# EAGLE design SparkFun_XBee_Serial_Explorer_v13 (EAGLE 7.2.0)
Assembly variants: Attributes
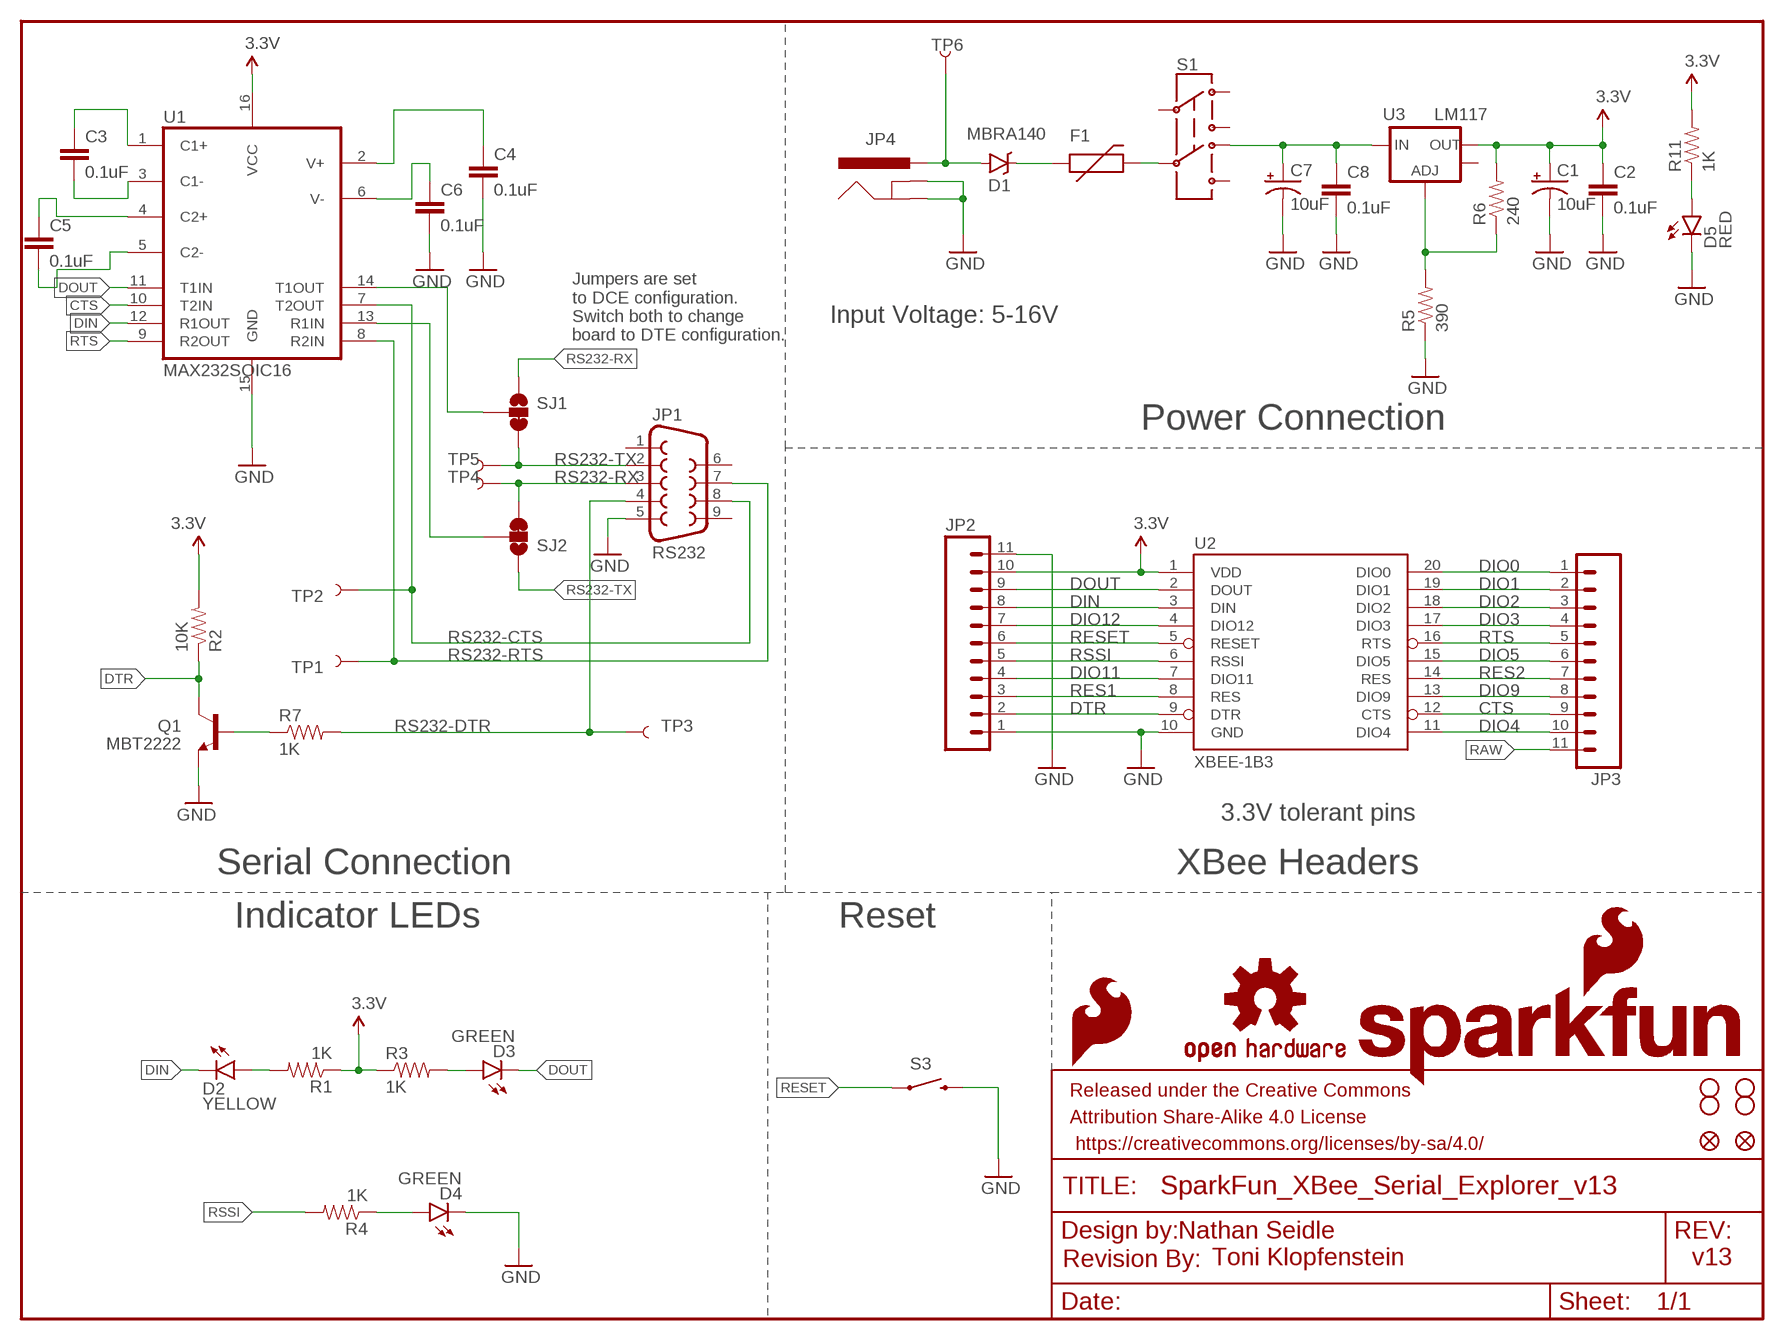
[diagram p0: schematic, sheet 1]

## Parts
C1  10uF  10UF-16V-10%(TANT)  [EIA3216]
C2  0.1uF  0.1UF-25V(+80/-20%)(0603)  [0603-CAP]
C3  0.1uF  0.1UF-25V(+80/-20%)(0603)  [0603-CAP]
C4  0.1uF  0.1UF-25V(+80/-20%)(0603)  [0603-CAP]
C5  0.1uF  0.1UF-25V(+80/-20%)(0603)  [0603-CAP]
C6  0.1uF  0.1UF-25V(+80/-20%)(0603)  [0603-CAP]
C7  10uF  10UF-16V-10%(TANT)  [EIA3216]
C8  0.1uF  0.1UF-25V(+80/-20%)(0603)  [0603-CAP]
D1  MBRA140  DIODE-SCHOTTKY-MBRA140  [SMA-DIODE]
D2  YELLOW  LED-YELLOWLARGE  [LED-1206]
D3  GREEN  LED-GREENLARGE  [LED-1206]
D4  GREEN  LED-GREENLARGE  [LED-1206]
D5  RED  LED-RED1206  [LED-1206]
F1  PTCTHERMISTOR1206  [PTC-1206]
FRAME1  FRAME-LETTER  [CREATIVE_COMMONS]
JP1  RS232  DB9FEMALE  [DB9]
JP2  M11PTH  [1X11]
JP3  M11PTH  [1X11]
JP4  POWER_JACKPTH_LOCK  [POWER_JACK_PTH_LOCK]
LOGO1  OSHW-LOGOL  [OSHW-LOGO-L]
LOGO2  SFE_LOGO_NAME_FLAME.2_INCH  [SFE_LOGO_NAME_FLAME_.2]
LOGO3  SFE_LOGO_FLAME.1_INCH  [SFE_LOGO_FLAME_.1]
Q1  MBT2222  TRANSISTOR_NPNSOT23-3  [SOT23-3]
R1  1K  1KOHM-1/10W-1%(0603)  [0603-RES]
R2  10K  10KOHM-1/10W-1%(0603)0603  [0603-RES]
R3  1K  1KOHM-1/10W-1%(0603)  [0603-RES]
R4  1K  1KOHM-1/10W-1%(0603)  [0603-RES]
R5  390  390OHM1/10W1%(0603)  [0603-RES]
R6  240  240OHM1/10W1%(0603)  [0603-RES]
R7  1K  1KOHM-1/10W-1%(0603)  [0603-RES]
R11  1K  1KOHM-1/10W-1%(0603)  [0603-RES]
S1  AYZ0202  [AYZ0202]
S3  TAC_SWITCHSMD  SWITCH-MOMENTARY-2SMD-REDUNDANT  [TACTILE-SWITCH-SMD]
SJ1  JUMPER-PAD-3-2OF3_NC_BY_TRACE_SMALL  [PAD-JUMPER-3-2OF3_NC_BY_TRACE_YES_SILK_FULL_BOX]
SJ2  JUMPER-PAD-3-2OF3_NC_BY_TRACE_SMALL  [PAD-JUMPER-3-2OF3_NC_BY_TRACE_YES_SILK_FULL_BOX]
TP1  TEST-POINTTP_15TH_THRU  [TP_15TH]
TP2  TEST-POINTTP_15TH_THRU  [TP_15TH]
TP3  TEST-POINTTP_15TH_THRU  [TP_15TH]
TP4  TEST-POINTTP_15TH_THRU  [TP_15TH]
TP5  TEST-POINTTP_15TH_THRU  [TP_15TH]
TP6  TEST-POINTTP_15TH_THRU  [TP_15TH]
U1  MAX232SOIC16  [SO016]
U2  XBEE-1B3  [XBEE-SMD]
U3  LM117  V_REG_LM1117SOT223  [SOT223]
U$1  REVISION  [REVISION]
U$5  STAND-OFF  [STAND-OFF]
U$7  FIDUCIAL1X2  [FIDUCIAL-1X2]
U$9  STAND-OFF  [STAND-OFF]
U$10  STAND-OFF  [STAND-OFF]
U$11  STAND-OFF  [STAND-OFF]
U$16  FIDUCIAL1X2  [FIDUCIAL-1X2]

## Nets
3.3V [vcc]: C1.A(+) C2.1 JP2.10 R1.1 R2.2 R3.1 R6.2 R11.2 U1.16(VCC) U2.1(VDD) U3.2(OUT)
CTS: JP3.9 U1.10(T2IN) U2.12(CTS)
DIN: D2.C JP2.8 U1.12(R1OUT) U2.3(DIN)
DIO0: JP3.1 U2.20(DIO0)
DIO1: JP3.2 U2.19(DIO1)
DIO2: JP3.3 U2.18(DIO2)
DIO3: JP3.4 U2.17(DIO3)
DIO4: JP3.10 U2.11(DIO4)
DIO5: JP3.6 U2.15(DIO5)
DIO9: JP3.8 U2.13(DIO9)
DIO11: JP2.4 U2.7(DIO11)
DIO12: JP2.7 U2.4(DIO12)
DOUT: D3.C JP2.9 U1.11(T1IN) U2.2(DOUT)
DTR: JP2.2 Q1.3(C) R2.1 U2.9(DTR)
GND [vcc]: C1.C(-) C2.2 C4.2 C6.2 C7.C(-) C8.2 D4.C D5.C JP1.5 JP2.1 JP2.11 JP4.GND JP4.GNDBREAK Q1.2(E) R5.1 S3.3 S3.4 U1.15(GND) U2.10(GND)
N$1: D2.A R1.2
N$2: D4.A R4.1
N$3: C3.1 U1.1(C1+)
N$4: D3.A R3.2
N$5: C3.2 U1.3(C1-)
N$6: C5.1 U1.4(C2+)
N$7: C5.2 U1.5(C2-)
N$8: C6.1 U1.6(V-)
N$9: C4.1 U1.2(V+)
N$10: R5.2 R6.1 U3.1(ADJ)
N$11: F1.2 S1.5
N$12: Q1.1(B) R7.1
N$13: SJ2.2 U1.13(R1IN)
N$14: SJ1.2 U1.14(T1OUT)
N$15: D1.A JP4.PWR TP6.P$1
N$16: D1.C F1.1
N$38: D5.A R11.1
RAW [vcc]: C7.A(+) C8.1 JP3.11 S1.6 U3.3(IN)
RES1: JP2.3 U2.8(RES)
RES2: JP3.7 U2.14(RES)
RESET: JP2.6 S3.1 S3.2 U2.5(RESET)
RS232-CTS: JP1.8 TP2.P$1 U1.7(T2OUT)
RS232-DTR: JP1.4 R7.2 TP3.P$1
RS232-RTS: JP1.7 TP1.P$1 U1.8(R2IN)
RS232-RX: JP1.3 SJ1.1 SJ2.3 TP4.P$1
RS232-TX: JP1.2 SJ1.3 SJ2.1 TP5.P$1
RSSI: JP2.5 R4.2 U2.6(RSSI)
RTS: JP3.5 U1.9(R2OUT) U2.16(RTS)
Unconnected: JP1.1 JP1.6 JP1.9 S1.1 S1.2 S1.3 S1.4 U3.4(OUT)

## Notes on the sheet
- Input Voltage: 5-16V
- Jumpers are set 
  to DCE configuration. 
  Switch both to change 
  board to DTE configuration.
- Power Connection
- 3.3V tolerant pins
- Serial Connection | XBee Headers
- Indicator LEDs | Reset
- Nathan Seidle
- Toni Klopfenstein | v13

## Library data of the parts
C1 C7 = SparkFun-Capacitors:10UF-16V-10%(TANT): CAP-00811; PROD_ID: CAP-00811
C2-C6 C8 = SparkFun-Capacitors:0.1UF-25V(+80/-20%)(0603): CAP-00810; PROD_ID: CAP-00810
D1 = SparkFun-DiscreteSemi:DIODE-SCHOTTKY: Schottky diodes in SFE's production catalog; PROD_ID: DIO-08053
D2 = SparkFun-LED:LED-YELLOW: Yellow SMD LEDs; PROD_ID: DIO-00820
D3 D4 = SparkFun-LED:LED-GREEN: Various green LEDs; PROD_ID: DIO-00862
D5 = SparkFun-LED:LED-RED: Assorted Red LEDs; PROD_ID: DIO-00809
F1 = SparkFun-PowerIC:PTC: Resettable Fuse PTC; PROD_ID: RES-08585
FRAME1 = SparkFun-Aesthetics:FRAME-LETTER: Schematic Frame
JP1 = SparkFun-Connectors:DB9: DB9 Connector Standard DB9 (D-Sub 9) serial connector. Can be used for CAN bus as well as RS485 and RS232. Footprint production proven. Spark Fun Electronics SKU : PRT-00429; PROD_ID: CONN-08194
JP2 JP3 = SparkFun:M11: Header 11 Standard 11-pin 0.1" header. Use with straight break away headers (SKU : PRT-00116), right angle break away headers (PRT-00553), swiss pins (PRT-00743), machine pins (PRT-00117), and female headers (PRT-00115).
JP4 = SparkFun-Connectors:POWER_JACK: Power Jack This is the standard 5.5mm barrel jack for power. The PTH is the most common, proven, reliable, footprint. The Slot footprint only works if the mill layer is transmitted to the PCB fab house so be warned. Mating wall wart : TOL-00298 (and others); PROD_ID: CONN-08197; SF_ID: PRT-00119
LOGO1 = SparkFun-Aesthetics:OSHW-LOGO: Open Source Hardware Logo This logo indicates the piece of hardware it is found on incorporates a OSHW license and/or adheres to the definition of open source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
LOGO2 = SparkFun-Aesthetics:SFE_LOGO_NAME_FLAME: SFE Logo, name and flame
LOGO3 = SparkFun-Aesthetics:SFE_LOGO_FLAME: SFE Logo, flame only
Q1 = SparkFun-DiscreteSemi:TRANSISTOR_NPN: Generic NPN BJT MMBT2222A - TRANS-08049 (SOT-23, 1A 40V) MPSA42 - TRANS-09116 (SOT-23, 500mA 300V) MMBT5088LT1G - TRANS-11160 (SOT-23, 50 mA 30V) BC547 - COM-08928 (TO-92 45V 100mA) (1.Collector 2.Base 3.Emitter) 2N3904 - COM-00521 (TO-92 40V 200mA) (1.Emitter 2.Base 3.Collector) P2N2222A -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; PROD_ID: TRANS-08049
R1 R3 R4 R7 R11 = SparkFun-Resistors:1KOHM-1/10W-1%(0603): RES-07856; PROD_ID: RES-07856
R2 = SparkFun-Resistors:10KOHM-1/10W-1%(0603): RES-00824; PROD_ID: RES-00824
R5 = SparkFun-Resistors:390OHM1/10W1%(0603): RES-07864; PROD_ID: RES-07864
R6 = SparkFun-Resistors:240OHM1/10W1%(0603): RES-07849; PROD_ID: RES-07849
S1 = SparkFun-Electromechanical:AYZ0202: SPDT Slide Switch Simple SMD single-pull double-throw slide switch. Good for less than 350mA power switch, switching UARTs between devices, etc. Spark Fun Electronics SKU : COM-00597; PROD_ID: SWCH-08179
S3 = SparkFun-Electromechanical:SWITCH-MOMENTARY-2: Various NO switches- pushbuttons, reed, etc; PROD_ID: SWCH-08247
SJ1 SJ2 = SparkFun-Passives:JUMPER-PAD-3-2OF3_NC_BY_TRACE
TP1-TP6 = SparkFun-Passives:TEST-POINT: Bare copper test points for troubleshooting or ICT
U1 = SparkFun-DigitalIC:MAX232: RS232 Transceiver Very common IC. This is generically called 'MAX232', but works with the 3V equivalent MAX3232 generic ICs. Field tested and mother approved. Spark Fun Electronics SKU : COM-00316 (DIP) and COM-00589 (SMD); PROD_ID: IC-08171
U2 = SparkFun-RF:XBEE-1: Xbee module footprints SMT header is CONN-09042.; PROD_ID: CONN-09042
U3 = SparkFun-PowerIC:V_REG_LM1117: Voltage Regulator LM1117 Standard adjustable voltage regulator but in SMD form. Spark Fun Electronics SKU : COM-00595; PROD_ID: VREG-08170
U$1 = SparkFun-Aesthetics:REVISION
U$5 U$9-U$11 = SparkFun-Electromechanical:STAND-OFF: #4 Stand Off
U$7 U$16 = SparkFun-Aesthetics:FIDUCIAL: Fiducial Alignment Points

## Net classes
0 default: width 0.203 mm
1 vcc: width 0.305 mm
2 gnd: width 0.254 mm

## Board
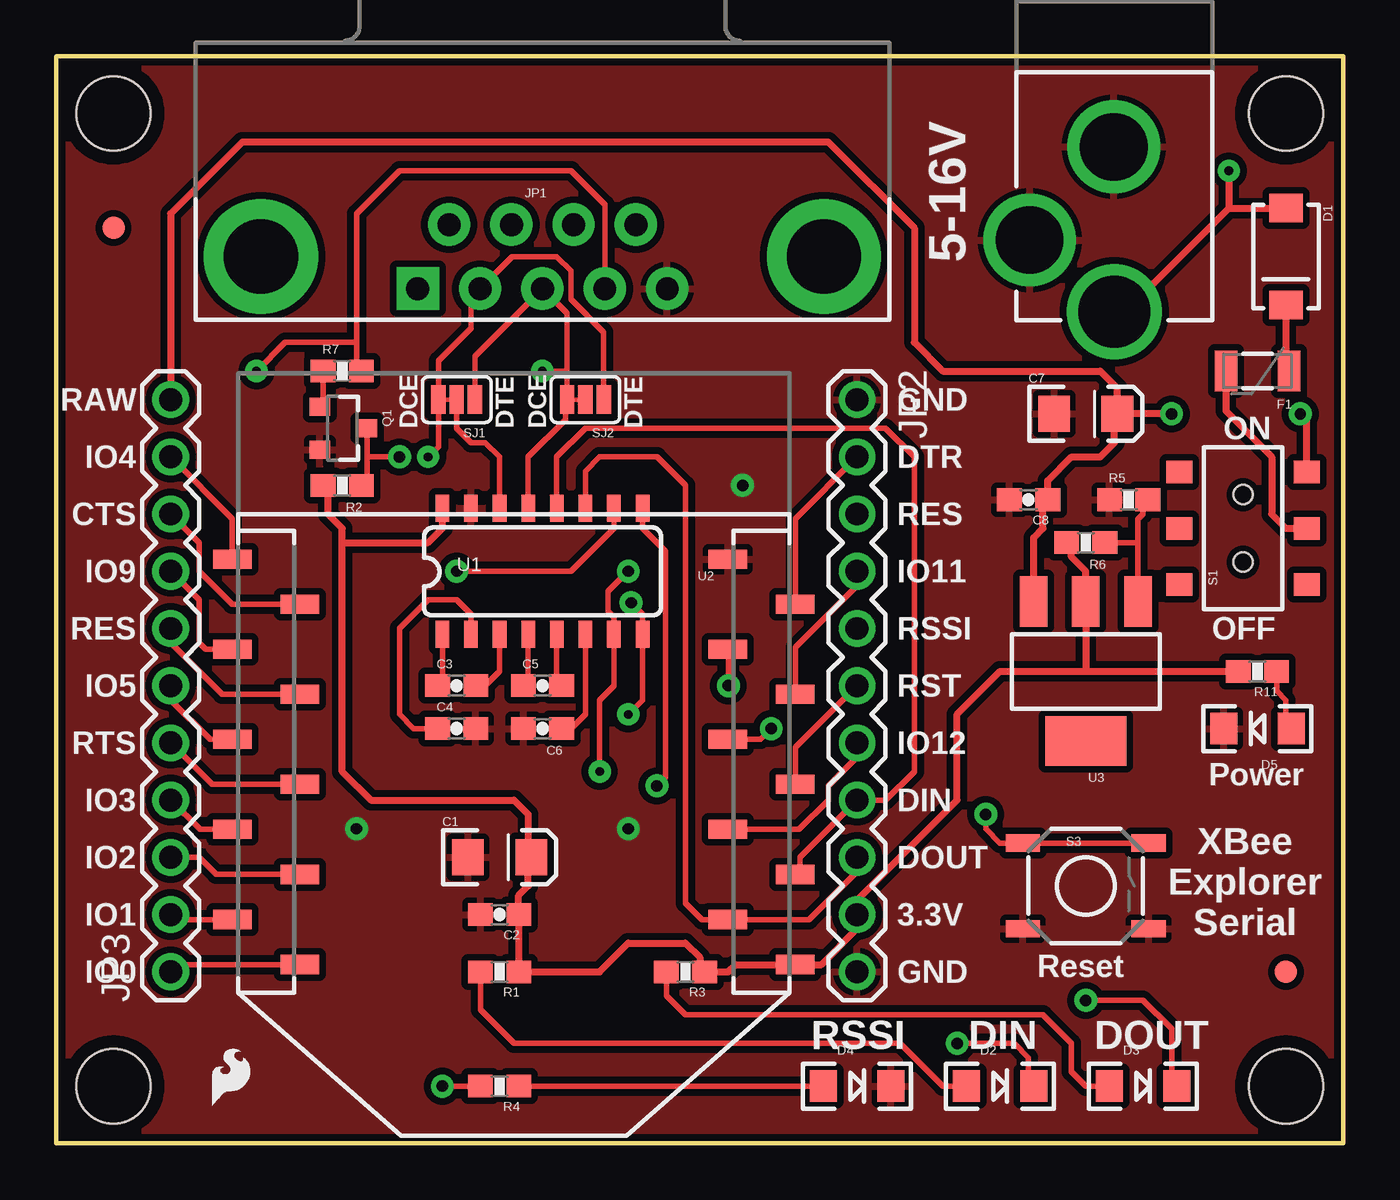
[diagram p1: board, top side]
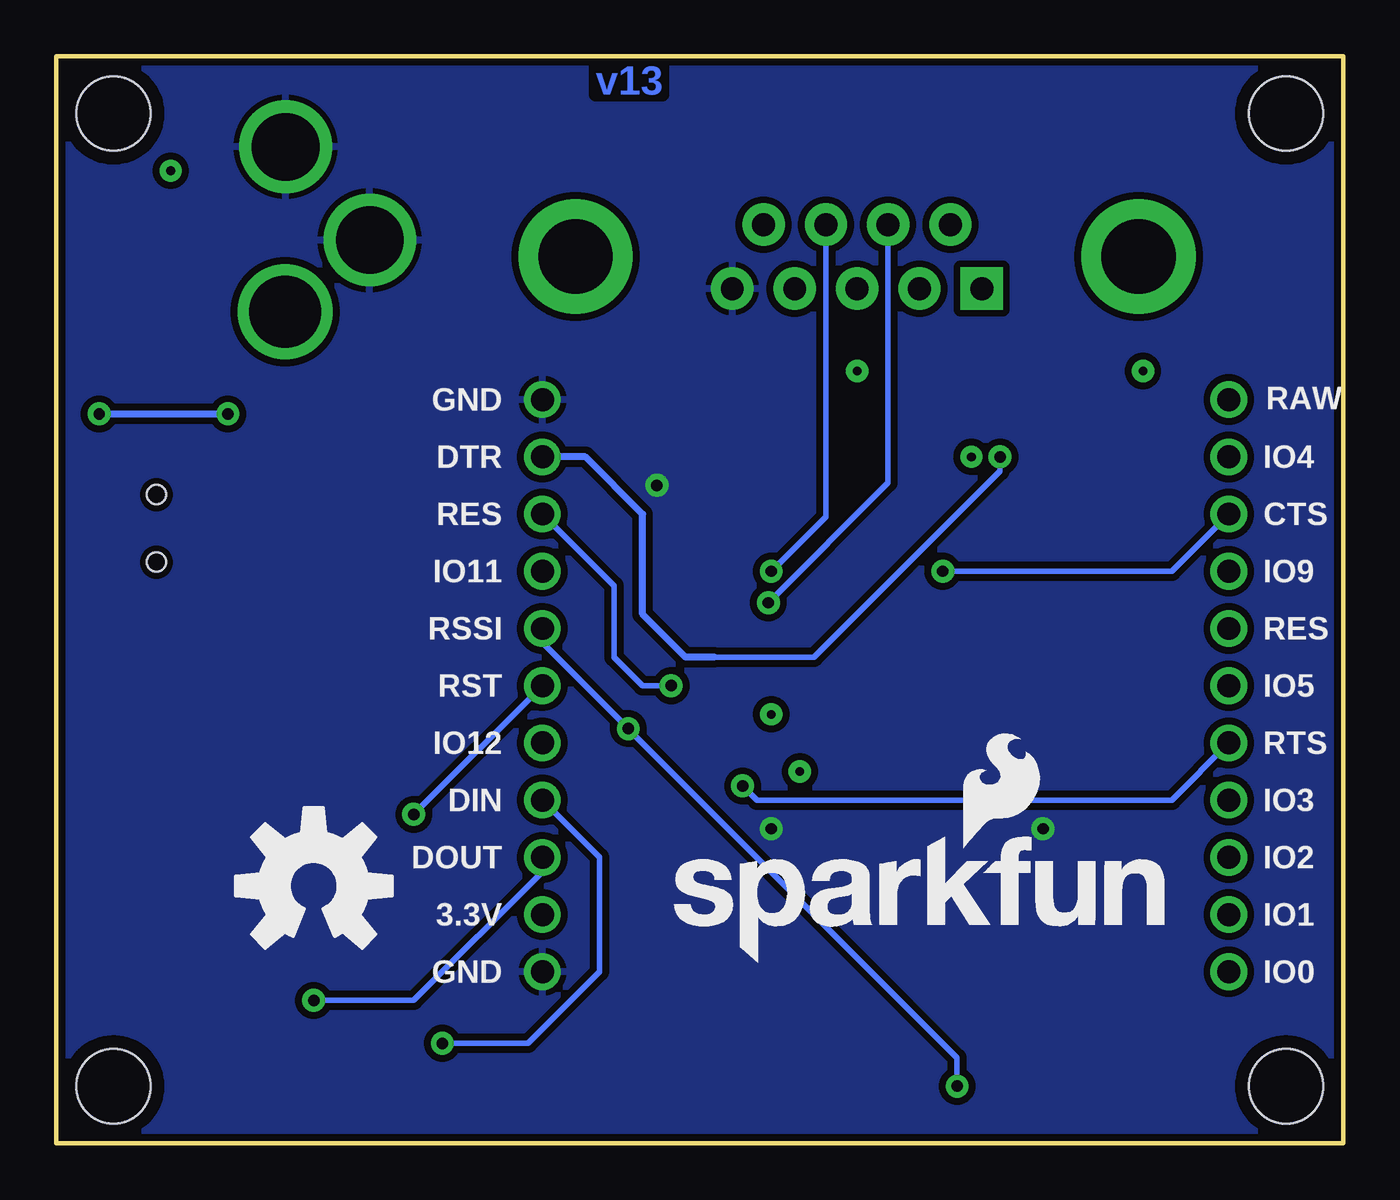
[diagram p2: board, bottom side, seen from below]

Size 57.15 x 48.26 mm. Coordinates in mm from the lower left corner, seen from the top.
Outline: 0,48.26 0,0 57.15,0 57.15,48.26 0,48.26
Copper layers (1*16): Top 0.035mm / dielectric 1.5mm / Bottom 0.035mm
Design rules "SparkFun-2-layer": minimum track width 7mil, minimum drill 15mil, track to track 8mil, track to pad 8mil, pad to pad 8mil, via to via 8mil, smd to smd 8mil, copper to edge 8mil, drill to drill 8mil, minimum pad ring 12mil, minimum via ring 10mil, stop-mask expansion 4mil, vias tented up to drill 20mil, thermal gap 10mil

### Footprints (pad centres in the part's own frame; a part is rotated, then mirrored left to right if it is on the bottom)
EIA3216 = smd 1.4 x 1.6: A 1.4,0; C -1.4,0
0603-CAP = smd 1.1 x 1: 1 -0.85,0; 2 0.85,0
SMA-DIODE = smd 1.27 x 1.47: A -2.15,0; C 2.15,0
LED-1206 = smd 1.2 x 1.4: A -1.5,0; C 1.5,0
PTC-1206 = smd 1 x 1.8: 1 -1.4,0; 2 1.4,0
DB9 = drill 1.016 pad 1.88 square: 1 -5.54,-1.42 | drill 1.016 pad 1.88: 2 -2.77,-1.42; 3 0,-1.42; 4 2.77,-1.42; 5 5.54,-1.42; 6 -4.15,1.42; 7 -1.38,1.42; 8 1.38,1.42; 9 4.15,1.42 | drill 3.302 pad 5.08: G1 -12.5,0; G2 12.5,0
1X11 = drill 1.016: 1 0,0; 2 2.54,0; 3 5.08,0; 4 7.62,0; 5 10.16,0; 6 12.7,0; 7 15.24,0; 8 17.78,0; 9 20.32,0; 10 22.86,0; 11 25.4,0
POWER_JACK_PTH_LOCK = drill 2.997 pad 4.115: GND 0.025,6.557; GNDBREAK 3.762,10.7 | drill 3.2 pad 4.115: PWR 0,13.878
SOT23-3 = smd 0.8 x 0.9: 1 -0.95,-1; 2 0.95,-1; 3 0,1.1
0603-RES = smd 1.1 x 1: 1 -0.85,0; 2 0.85,0
AYZ0202 = smd 1 x 1.15: 1 -2.5,2.825; 2 0,2.825; 3 2.5,2.825; 4 -2.5,-2.825; 5 0,-2.825; 6 2.5,-2.825 | hole 0.85: 1.5,0; -1.5,0
TACTILE-SWITCH-SMD = smd 1.524 x 0.762: 1 -2.794,1.905; 2 2.794,1.905; 3 -2.794,-1.905; 4 2.794,-1.905
PAD-JUMPER-3-2OF3_NC_BY_TRACE_YES_SILK_FULL_BOX = smd 0.635 x 1.27: 1 -0.813,0; 2 0,0; 3 0.813,0
TP_15TH = drill 0.381 pad 0.61: P$1 0,0
SO016 = smd 0.6 x 1.2: 1 -4.445,-2.8; 2 -3.175,-2.8; 3 -1.905,-2.8; 4 -0.635,-2.8; 5 0.635,-2.8; 6 1.905,-2.8; 7 3.175,-2.8; 8 4.445,-2.8; 9 4.445,2.8; 10 3.175,2.8; 11 1.905,2.8; 12 0.635,2.8; 13 -0.635,2.8; 14 -1.905,2.8; 15 -3.175,2.8; 16 -4.445,2.8
XBEE-SMD = smd 1.7 x 0.85: 1 -12.5,20; 2 -9.5,18; 3 -12.5,16; 4 -9.5,14; 5 -12.5,12; 6 -9.5,10; 7 -12.5,8; 8 -9.5,6; 9 -12.5,4; 10 -9.5,2; 11 12.5,2; 12 9.5,4; 13 12.5,6; 14 9.5,8; 15 12.5,10; 16 9.5,12; 17 12.5,14; 18 9.5,16; 19 12.5,18; 20 9.5,20
SOT223 = smd 1.219 x 2.235: 1 -2.311,-3.099; 2 0,-3.099; 3 2.311,-3.099 | smd 3.6 x 2.2: 4 0,3.099
STAND-OFF = hole 3.302: 0,0
FIDUCIAL-1X2 = smd 1 x 1: 1 0,0

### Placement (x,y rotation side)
C1  19.68,12.7 0 top
C2  19.68,10.16 180 top
C3  17.78,20.32 0 top
C4  17.78,18.41 0 top
C5  21.59,20.32 0 top
C6  21.59,18.41 180 top
C7  45.72,32.38 0 top
C8  43.18,28.57 180 top
D1  54.61,39.37 270 top
D2  41.91,2.54 0 top
D3  48.26,2.54 0 top
D4  35.56,2.54 0 top
D5  53.34,18.41 180 top
F1  53.34,34.29 180 top
FRAME1  not placed on the board
JP1  21.59,39.37 0 top
JP2  35.56,33.02 270 top
JP3  5.08,7.62 90 top
JP4  46.99,50.8 180 top
LOGO1  45.72,11.43 0 bottom
LOGO2  30.43,7.92 0 bottom
LOGO3  6.6,1.32 0 top
Q1  12.7,31.75 270 top
R1  19.68,7.62 180 top
R2  12.7,29.21 180 top
R3  27.94,7.62 180 top
R4  19.68,2.54 180 top
R5  47.62,28.57 0 top
R6  45.72,26.67 180 top
R7  12.7,34.29 0 top
R11  53.34,20.95 180 top
S1  52.7,27.3 90 top
S3  45.72,11.43 0 top
SJ1  17.78,33.02 180 top
SJ2  23.5,33.02 180 top
TP1  25.4,19.05 0 top
TP2  24.13,16.51 0 top
TP3  8.89,34.29 0 top
TP4  21.59,34.29 0 top
TP5  16.51,30.48 0 top
TP6  52.07,43.18 0 top
U1  21.59,25.4 0 top
U2  20.32,27.94 180 top
U3  45.72,20.95 180 top
U$1  not placed on the board
U$5  2.54,2.54 270 top
U$7  2.54,40.64 270 top
U$9  54.61,2.54 270 top
U$10  54.61,45.72 270 top
U$11  2.54,45.72 270 top
U$16  54.61,7.62 270 top

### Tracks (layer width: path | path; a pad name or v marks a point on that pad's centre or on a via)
3.3V
  Top 0.305: 12.7,26.67 16.51,26.67 17.14,27.3 U1.16 | 12.7,26.67 12.7,16.51 13.97,15.24 20.32,15.24 20.95,14.61 20.95,12.83 C1.A 20.95,12.57 20.95,11.43 20.54,11.01 C2.1 R1.1 24.13,7.62 25.4,8.89 27.94,8.89 28.57,8.26 28.57,7.83 R3.1 29.84,7.62 30.16,7.94 U2.1 33.98,7.94 35.56,9.53 JP2.10 35.56,10.79 40.01,15.24 40.01,19.05 41.91,20.95 45.72,20.95 | 12.7,26.67 12.7,27.3 12.06,27.94 12.06,29 R2.2 | 45.72,20.95 R11.2 | 45.72,20.95 U3.2 45.72,25.4 45.09,26.04 45.09,26.45 R6.2
CTS  (via drill 0.51)
  Top 0.254: U1.10 24.77,27.3 22.86,25.4 v17.78,25.4 | U2.12 7.81,23.94 6.35,25.4 6.35,26.67 JP3.9
  Bottom 0.254: v17.78,25.4 7.62,25.4 JP3.9
DIN  (via drill 0.51)
  Top 0.254: U2.3 33.02,11.94 33.02,12.7 JP2.8 36.83,15.24 38.1,16.51 38.1,30.48 36.83,31.75 23.5,31.75 22.23,30.48 U1.12 22.23,28.7 22.35,28.57 | v40.01,4.45 42.55,4.45 43.18,3.81 43.18,2.77 D2.C
  Bottom 0.254: JP2.8 33.02,12.7 33.02,7.62 36.2,4.45 v40.01,4.45
DIO0
  Top 0.254: U2.20 5.4,7.94 JP3.1
DIO1
  Top 0.254: U2.19 5.3,9.94 JP3.2
DIO2
  Top 0.254: U2.18 7.11,11.94 6.35,12.7 JP3.3
DIO3
  Top 0.254: U2.17 6.38,13.94 JP3.4
DIO4
  Top 0.254: U2.11 7.82,27.74 JP3.10
DIO5
  Top 0.254: U2.15 6.83,17.94 5.08,19.68 JP3.6
DIO9
  Top 0.254: U2.13 6.63,21.94 6.35,22.23 6.35,24.13 JP3.8
DIO11
  Top 0.254: U2.7 32.82,22.02 35.56,24.77 JP2.4
DIO12
  Top 0.254: U2.4 32.99,13.94 34.29,15.24 34.29,15.88 35.56,17.14 JP2.7
DOUT  (via drill 0.51)
  Top 0.254: U1.11 23.5,29.84 24.13,30.48 26.67,30.48 27.94,29.21 27.94,10.67 28.67,9.94 U2.2 33.44,9.94 35.56,12.06 JP2.9 | v45.72,6.35 48.26,6.35 49.53,5.08 49.53,2.77 D3.C
  Bottom 0.254: JP2.9 35.56,12.06 41.27,6.35 v45.72,6.35
DTR  (via drill 0.51)
  Top 0.254: U2.9 32.82,27.74 JP2.2 | Q1.3 13.8,30.48 | 13.8,30.48 13.8,29.46 R2.1 | v15.24,30.48 13.8,30.48
  Bottom 0.254: 27.94,21.59 23.5,21.59 15.24,29.84 v15.24,30.48
  Bottom 0.305: 27.94,21.59 29.21,21.59 31.11,23.5 31.11,27.94 33.66,30.48 JP2.2
GND  (via drill 0.51)
  other vias: 30.48,29.21 25.4,13.97 13.34,13.97
  pour Bottom (isolate 0.305): 57.15,48.26 57.15,0 0,0 0,48.26
  pour Top (isolate 0.305): 57.15,48.26 57.15,0 0,0 0,48.26
N$1
  Top 0.254: D2.A 39.37,2.54 37.47,4.45 20.32,4.45 18.84,5.93 R1.2
N$2
  Top 0.254: R4.1 D4.A
N$3
  Top 0.254: U1.1 17.14,20.54 C3.1
N$4
  Top 0.254: D3.A 45.72,2.54 45.09,3.17 45.09,4.45 43.81,5.71 27.94,5.71 27.09,6.57 R3.2
N$5
  Top 0.254: U1.3 19.68,20.95 19.05,20.32 C3.2
N$6
  Top 0.254: U1.4 20.95,20.54 C5.1
N$7
  Top 0.254: U1.5 22.23,20.54 C5.2
N$8
  Top 0.254: C6.1 22.86,18.41 23.5,19.05 U1.6
N$9
  Top 0.254: U1.2 18.41,23.5 17.78,24.13 16.51,24.13 15.24,22.86 15.24,19.05 15.88,18.41 C4.1
N$10
  Top 0.254: U3.1 48.03,26.67 | 48.03,26.67 48.03,27.71 48.26,27.94 48.26,28.36 R5.2 | R6.1 48.03,26.67
N$11
  Top 0.305: F1.2 51.94,32.52 53.98,30.48 53.98,27.94 54.61,27.3 S1.5
N$12
  Top 0.254: R7.1 11.85,32.85 Q1.1
N$13
  Top 0.254: U1.13 20.95,30.48 22.61,32.13 22.61,32.77 22.86,33.02
N$14
  Top 0.254: U1.14 19.68,30.48 19.05,31.11 18.41,31.11 17.78,31.75 SJ1.2
N$15
  Top 0.305: TP6.P$1 52.07,41.52 | JP4.PWR 47.47,36.92 52.07,41.52 | 52.07,41.52 D1.A
N$16
  Top 0.305: D1.C 54.61,34.42 F1.1
N$38
  Top 0.254: R11.1 54.19,20.11 54.61,19.68 54.61,18.64 D5.A
RAW  (via drill 0.51)
  Top 0.305: JP3.11 5.08,41.27 8.26,44.45 34.29,44.45 38.1,40.64 38.1,35.56 39.37,34.29 46.35,34.29 47.12,33.52 C7.A | v49.53,32.38 C7.A | U3.3 43.41,26.9 43.81,27.3 43.81,28.36 C8.1 44.03,29.43 45.09,30.48 46.35,30.48 46.99,31.11 46.99,32.26 C7.A | S1.6 55.53,32.1 v55.24,32.38
  Bottom 0.305: v55.24,32.38 v49.53,32.38
RES1  (via drill 0.51)
  Top 0.254: U2.8 29.84,21.91 v29.84,20.32
  Bottom 0.254: JP2.3 32.38,24.77 32.38,21.59 31.11,20.32 v29.84,20.32
RES2
  Top 0.254: U2.14 7.37,19.94 5.08,22.23 JP3.7
RESET  (via drill 0.51)
  Top 0.254: v41.27,14.61 41.27,13.97 41.91,13.34 S3.1 S3.2 48.9,13.34 | U2.5 32.82,17.58 JP2.6
  Bottom 0.254: JP2.6 v41.27,14.61
RS232-CTS  (via drill 0.51)
  Top 0.254: v25.4,25.4 24.51,24.51 24.51,23.62 24.77,23.37 U1.7 24.77,20.32 24.13,19.68 TP2.P$1
  Bottom 0.254: JP1.8 22.97,27.83 v25.4,25.4
RS232-DTR
  Top 0.254: JP1.4 24.36,41.68 22.86,43.18 15.24,43.18 13.34,41.27 13.34,35.56 | 13.34,35.56 13.34,34.51 R7.2 | TP3.P$1 10.16,35.56 13.34,35.56
RS232-RTS  (via drill 0.51)
  Top 0.254: v25.53,24 26.04,23.5 U1.8 26.04,19.68 TP1.P$1
  Bottom 0.254: v25.53,24 20.21,29.32 JP1.7
RS232-RX
  Top 0.254: SJ1.1 18.59,34.95 JP1.3 22.68,36.86 22.68,34.29 | SJ2.3 22.68,34.29 | TP4.P$1 22.68,34.29
RS232-TX
  Top 0.254: SJ2.1 24.31,36.02 22.86,37.47 22.86,38.73 22.23,39.37 20.24,39.37 JP1.2 18.41,37.55 18.41,36.2 16.97,34.75 SJ1.3 16.97,30.94 TP5.P$1
RSSI  (via drill 0.51)
  Top 0.254: R4.2 v17.14,2.54 | U2.6 31.27,17.94 v31.75,18.41
  Bottom 0.254: JP2.5 35.56,22.23 32.07,18.73 v31.75,18.41 17.14,3.81 v17.14,2.54
RTS  (via drill 0.51)
  Top 0.254: 10.79,15.75 10.82,15.77 U2.16 6.92,15.94 JP3.5 | U1.9 26.04,27.3 27.05,26.29 27.05,16.26 v26.67,15.88
  Bottom 0.254: JP3.5 7.62,15.24 26.04,15.24 v26.67,15.88

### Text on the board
Bottom: v13
tPlace: 5-16V | RAW | GND | DCE | DTE | DCE | DTE | ON | IO4 | DTR | CTS | RES | IO9 | IO11 | RES | RSSI | OFF | IO5 | RST | RTS | IO12 | Power | IO3 | DIN | XBee / Explorer / Serial | IO2 | DOUT | IO1 | 3.3V | IO0 | GND | Reset | RSSI | DIN | DOUT
bPlace: RAW | GND | IO4 | DTR | CTS | RES | IO9 | IO11 | RES | RSSI | IO5 | RST | RTS | IO12 | IO3 | DIN | IO2 | DOUT | IO1 | 3.3V | IO0 | GND
tDocu: Nathan Seidle | Toni Klopfenstein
